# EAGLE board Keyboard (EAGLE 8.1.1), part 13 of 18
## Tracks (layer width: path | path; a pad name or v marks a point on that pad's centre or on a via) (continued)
S$13256 (continued)
  Bottom 0: 115.9,40.92 115.77,41.25
S$13257
  Bottom 0: 115.77,41.25 115.57,41.53
S$13258
  Bottom 0: 115.57,41.53 115.3,41.76
S$13259
  Bottom 0: 115.3,41.76 114.98,41.91
S$13260
  Bottom 0: 114.98,41.91 114.64,41.97
S$13261
  Bottom 0: 114.64,41.97 114.29,41.95
S$13262
  Bottom 0: 114.29,41.95 113.96,41.84
S$13263
  Bottom 0: 113.96,41.84 113.93,41.83
S$13264
  Bottom 0: 113.93,41.83 113.36,42.4
S$13265
  Bottom 0: 113.36,42.4 113.31,42.43
S$13266
  Bottom 0: 113.31,42.43 113.25,42.48
S$13267
  Bottom 0: 113.25,42.48 113.19,42.5
S$13268
  Bottom 0: 113.19,42.5 113.12,42.52
S$13269
  Bottom 0: 113.12,42.52 113.05,42.52
S$13270
  Bottom 0: 113.05,42.52 108.48,42.52
S$13271
  Bottom 0: 108.48,42.52 108.42,42.65
S$13272
  Bottom 0: 108.42,42.65 108.21,42.87
S$13273
  Bottom 0: 108.21,42.87 107.95,43.02
S$13274
  Bottom 0: 107.95,43.02 107.65,43.09
S$13275
  Bottom 0: 107.65,43.09 107.35,43.07
S$13276
  Bottom 0: 107.35,43.07 107.07,42.96
S$13277
  Bottom 0: 107.07,42.96 106.83,42.77
S$13278
  Bottom 0: 106.83,42.77 106.66,42.52
S$13279
  Bottom 0: 106.66,42.52 106.57,42.23
S$13280
  Bottom 0: 106.57,42.23 106.57,41.92
S$13281
  Bottom 0: 106.57,41.92 106.66,41.64
S$13282
  Bottom 0: 106.66,41.64 106.83,41.39
S$13283
  Bottom 0: 106.83,41.39 107.07,41.2
S$13284
  Bottom 0: 107.07,41.2 107.35,41.09
S$13285
  Bottom 0: 107.35,41.09 107.65,41.07
S$13286
  Bottom 0: 107.65,41.07 107.95,41.13
S$13287
  Bottom 0: 107.95,41.13 108.21,41.28
S$13288
  Bottom 0: 108.21,41.28 108.42,41.51
S$13289
  Bottom 0: 108.42,41.51 108.48,41.64
S$13290
  Bottom 0: 108.48,41.64 112.86,41.64
S$13291
  Bottom 0: 112.86,41.64 113.31,41.19
S$13292
  Bottom 0: 113.31,41.19 113.25,41.09
S$13293
  Bottom 0: 113.25,41.09 113.17,40.75
S$13294
  Bottom 0: 113.17,40.75 113.17,40.4
S$13295
  Bottom 0: 113.17,40.4 113.25,40.06
S$13296
  Bottom 0: 113.25,40.06 113.42,39.75
S$13297
  Bottom 0: 113.42,39.75 113.66,39.5
S$13298
  Bottom 0: 113.66,39.5 113.96,39.31
S$13299
  Bottom 0: 113.96,39.31 114.29,39.2
S$13300
  Bottom 0: 114.29,39.2 114.64,39.19
S$13301
  Bottom 0: 114.64,39.19 114.84,39.22
S$13302
  Bottom 0: 114.84,39.22 112.44,36.82
S$13303
  Bottom 0: 112.44,36.82 110.82,36.82
S$13304
  Bottom 0: 110.82,36.82 110.75,36.82
S$13305
  Bottom 0: 110.75,36.82 110.69,36.8
S$13306
  Bottom 0: 110.69,36.8 110.62,36.78
S$13307
  Bottom 0: 110.62,36.78 110.56,36.74
S$13308
  Bottom 0: 110.56,36.74 110.51,36.7
S$13309
  Bottom 0: 110.51,36.7 107.24,33.43
S$13310
  Bottom 0: 107.24,33.43 107.2,33.37
S$13311
  Bottom 0: 107.2,33.37 107.16,33.31
S$13312
  Bottom 0: 107.16,33.31 107.14,33.25
S$13313
  Bottom 0: 107.14,33.25 107.12,33.19
S$13314
  Bottom 0: 107.12,33.19 107.11,33.11
S$13315
  Bottom 0: 107.11,33.11 107.11,32.83
S$13316
  Bottom 0: 107.11,32.83 106.74,32.83
S$13317
  Bottom 0: 106.74,32.83 106.74,32.96
S$13318
  Bottom 0: 106.74,32.96 106.68,33.18
S$13319
  Bottom 0: 106.68,33.18 106.52,33.34
S$13320
  Bottom 0: 106.52,33.34 106.3,33.4
S$13321
  Bottom 0: 106.3,33.4 105.95,33.4
S$13322
  Bottom 0: 105.95,33.4 104.86,34.49
S$13323
  Bottom 0: 104.86,34.49 104.92,34.62
S$13324
  Bottom 0: 104.92,34.62 104.97,34.94
S$13325
  Bottom 0: 104.97,34.94 104.92,35.26
S$13326
  Bottom 0: 104.92,35.26 104.79,35.56
S$13327
  Bottom 0: 104.79,35.56 104.58,35.82
S$13328
  Bottom 0: 104.58,35.82 104.32,36.01
S$13329
  Bottom 0: 104.32,36.01 104.02,36.11
S$13330
  Bottom 0: 104.02,36.11 103.69,36.13
S$13331
  Bottom 0: 103.69,36.13 103.37,36.06
S$13332
  Bottom 0: 103.37,36.06 103.08,35.92
S$13333
  Bottom 0: 103.08,35.92 102.85,35.7
S$13334
  Bottom 0: 102.85,35.7 102.67,35.42
S$13335
  Bottom 0: 102.67,35.42 102.59,35.1
S$13336
  Bottom 0: 102.59,35.1 102.59,34.78
S$13337
  Bottom 0: 102.59,34.78 102.67,34.47
S$13338
  Bottom 0: 102.67,34.47 102.85,34.19
S$13339
  Bottom 0: 102.85,34.19 103.08,33.97
S$13340
  Bottom 0: 103.08,33.97 103.37,33.82
S$13341
  Bottom 0: 103.37,33.82 103.69,33.75
S$13342
  Bottom 0: 103.69,33.75 104.02,33.77
S$13343
  Bottom 0: 104.02,33.77 104.23,33.85
S$13344
  Bottom 0: 104.23,33.85 105.29,32.79
S$13345
  Bottom 0: 105.29,32.79 105.26,32.78
S$13346
  Bottom 0: 105.26,32.78 105.21,32.72
S$13347
  Bottom 0: 105.21,32.72 105.17,32.65
S$13348
  Bottom 0: 105.17,32.65 105.16,32.58
S$13349
  Bottom 0: 105.16,32.58 105.16,30.8
S$13350
  Bottom 0: 105.16,30.8 105.17,30.72
S$13351
  Bottom 0: 105.17,30.72 105.21,30.65
S$13352
  Bottom 0: 105.21,30.65 105.26,30.59
S$13353
  Bottom 0: 105.26,30.59 105.34,30.55
S$13354
  Bottom 0: 105.34,30.55 105.41,30.54
S$13355
  Bottom 0: 105.41,30.54 106.93,30.54
S$13356
  Bottom 0: 106.93,30.54 104.68,28.29
S$13357
  Bottom 0: 104.68,28.29 104.44,28.27
S$13358
  Bottom 0: 104.44,28.27 104.22,28.16
S$13359
  Bottom 0: 104.22,28.16 104.05,27.97
S$13360
  Bottom 0: 104.05,27.97 103.95,27.74
S$13361
  Bottom 0: 103.95,27.74 103.95,27.48
S$13362
  Bottom 0: 103.95,27.48 104.05,27.25
S$13363
  Bottom 0: 104.05,27.25 104.22,27.06
S$13364
  Bottom 0: 104.22,27.06 104.44,26.95
S$13365
  Bottom 0: 104.44,26.95 104.69,26.93
S$13366
  Bottom 0: 104.69,26.93 104.94,27
S$13367
  Bottom 0: 104.94,27 105.14,27.15
S$13368
  Bottom 0: 105.14,27.15 105.27,27.36
S$13369
  Bottom 0: 105.27,27.36 105.32,27.61
S$13370
  Bottom 0: 105.32,27.61 105.31,27.66
S$13371
  Bottom 0: 105.31,27.66 107.87,30.22
S$13372
  Bottom 0: 107.87,30.22 107.91,30.28
S$13373
  Bottom 0: 107.91,30.28 107.95,30.34
S$13374
  Bottom 0: 107.95,30.34 107.98,30.4
S$13375
  Bottom 0: 107.98,30.4 107.99,30.47
S$13376
  Bottom 0: 107.99,30.47 108,30.54
S$13377
  Bottom 0: 108,30.54 108,30.93
S$13378
  Bottom 0: 108,30.93 108.09,30.82
S$13379
  Bottom 0: 108.09,30.82 108.37,30.64
S$13380
  Bottom 0: 108.37,30.64 108.68,30.55
S$13381
  Bottom 0: 108.68,30.55 109,30.55
S$13382
  Bottom 0: 109,30.55 109.31,30.64
S$13383
  Bottom 0: 109.31,30.64 109.59,30.82
S$13384
  Bottom 0: 109.59,30.82 109.8,31.07
S$13385
  Bottom 0: 109.8,31.07 109.94,31.37
S$13386
  Bottom 0: 109.94,31.37 109.98,31.69
S$13387
  Bottom 0: 109.98,31.69 109.94,32.01
S$13388
  Bottom 0: 109.94,32.01 109.8,32.31
S$13389
  Bottom 0: 109.8,32.31 109.59,32.55
S$13390
  Bottom 0: 109.59,32.55 109.31,32.73
S$13391
  Bottom 0: 109.31,32.73 109,32.82
S$13392
  Bottom 0: 109,32.82 108.68,32.82
S$13393
  Bottom 0: 108.68,32.82 108.37,32.73
S$13394
  Bottom 0: 108.37,32.73 108.09,32.55
S$13395
  Bottom 0: 108.09,32.55 108,32.44
S$13396
  Bottom 0: 108,32.44 108,32.93
S$13397
  Bottom 0: 108,32.93 110.22,35.15
S$13398
  Bottom 0: 110.22,35.15 110.21,35.1
S$13399
  Bottom 0: 110.21,35.1 110.21,34.78
S$13400
  Bottom 0: 110.21,34.78 110.29,34.47
S$13401
  Bottom 0: 110.29,34.47 110.47,34.19
S$13402
  Bottom 0: 110.47,34.19 110.7,33.97
S$13403
  Bottom 0: 110.7,33.97 110.82,33.91
S$13404
  Bottom 0: 110.82,33.91 110.82,26.95
S$13405
  Bottom 0: 110.82,26.95 109.72,25.85
S$13406
  Bottom 0: 107.65,48.69 107.95,48.76
S$13407
  Bottom 0: 107.95,48.76 108.21,48.91
S$13408
  Bottom 0: 108.21,48.91 108.42,49.13
S$13409
  Bottom 0: 108.42,49.13 108.55,49.4
S$13410
  Bottom 0: 108.55,49.4 108.59,49.7
S$13411
  Bottom 0: 108.59,49.7 108.55,50
S$13412
  Bottom 0: 108.55,50 108.42,50.27
S$13413
  Bottom 0: 108.42,50.27 108.21,50.49
S$13414
  Bottom 0: 108.21,50.49 107.95,50.65
S$13415
  Bottom 0: 107.95,50.65 107.65,50.71
S$13416
  Bottom 0: 107.65,50.71 107.35,50.69
S$13417
  Bottom 0: 107.35,50.69 107.07,50.58
S$13418
  Bottom 0: 107.07,50.58 106.83,50.39
S$13419
  Bottom 0: 106.83,50.39 106.66,50.14
S$13420
  Bottom 0: 106.66,50.14 106.57,49.85
S$13421
  Bottom 0: 106.57,49.85 106.57,49.55
S$13422
  Bottom 0: 106.57,49.55 106.66,49.26
S$13423
  Bottom 0: 106.66,49.26 106.83,49.01
S$13424
  Bottom 0: 106.83,49.01 107.07,48.82
S$13425
  Bottom 0: 107.07,48.82 107.35,48.71
S$13426
  Bottom 0: 107.35,48.71 107.65,48.69
S$13427
  Bottom 0: 147.88,27.16 147.78,27.48
S$13428
  Bottom 0: 147.78,27.48 147.57,27.88
S$13429
  Bottom 0: 147.57,27.88 147.28,28.22
S$13430
  Bottom 0: 147.28,28.22 146.94,28.51
S$13431
  Bottom 0: 146.94,28.51 146.54,28.72
S$13432
  Bottom 0: 146.54,28.72 146.11,28.85
S$13433
  Bottom 0: 146.11,28.85 145.67,28.89
S$13434
  Bottom 0: 145.67,28.89 145.22,28.85
S$13435
  Bottom 0: 145.22,28.85 144.79,28.72
S$13436
  Bottom 0: 144.79,28.72 144.74,28.69
S$13437
  Bottom 0: 144.74,28.69 146.64,30.59
S$13438
  Bottom 0: 146.64,30.59 146.77,30.55
S$13439
  Bottom 0: 146.77,30.55 147.1,30.55
S$13440
  Bottom 0: 147.1,30.55 147.41,30.64
S$13441
  Bottom 0: 147.41,30.64 147.68,30.82
S$13442
  Bottom 0: 147.68,30.82 147.88,31.04
S$13443
  Bottom 0: 147.88,31.04 147.88,27.16
S$13444
  Bottom 0: 142.43,27.99 138.07,32.35
S$13445
  Bottom 0: 138.07,32.35 138.01,32.41
S$13446
  Bottom 0: 138.01,32.41 137.93,32.45
S$13447
  Bottom 0: 137.93,32.45 137.85,32.49
S$13448
  Bottom 0: 137.85,32.49 137.76,32.51
S$13449
  Bottom 0: 137.76,32.51 137.67,32.52
S$13450
  Bottom 0: 137.67,32.52 128.66,32.52
S$13451
  Bottom 0: 128.66,32.52 128.63,32.55
S$13452
  Bottom 0: 128.63,32.55 128.36,32.73
S$13453
  Bottom 0: 128.36,32.73 128.05,32.82
S$13454
  Bottom 0: 128.05,32.82 127.72,32.82
S$13455
  Bottom 0: 127.72,32.82 127.41,32.73
S$13456
  Bottom 0: 127.41,32.73 127.14,32.55
S$13457
  Bottom 0: 127.14,32.55 126.93,32.31
S$13458
  Bottom 0: 126.93,32.31 126.79,32.01
S$13459
  Bottom 0: 126.79,32.01 126.74,31.69
S$13460
  Bottom 0: 126.74,31.69 126.79,31.37
S$13461
  Bottom 0: 126.79,31.37 126.93,31.07
S$13462
  Bottom 0: 126.93,31.07 127.14,30.82
S$13463
  Bottom 0: 127.14,30.82 127.32,30.71
S$13464
  Bottom 0: 127.32,30.71 126.47,30.71
S$13465
  Bottom 0: 126.47,30.71 126.48,30.72
S$13466
  Bottom 0: 126.48,30.72 126.49,30.8
S$13467
  Bottom 0: 126.49,30.8 126.49,32.58
S$13468
  Bottom 0: 126.49,32.58 126.48,32.65
S$13469
  Bottom 0: 126.48,32.65 126.44,32.72
S$13470
  Bottom 0: 126.44,32.72 126.38,32.78
S$13471
  Bottom 0: 126.38,32.78 126.31,32.82
S$13472
  Bottom 0: 126.31,32.82 126.23,32.83
S$13473
  Bottom 0: 126.23,32.83 125.79,32.83
S$13474
  Bottom 0: 125.79,32.83 125.79,32.96
S$13475
  Bottom 0: 125.79,32.96 125.73,33.18
S$13476
  Bottom 0: 125.73,33.18 125.56,33.34
S$13477
  Bottom 0: 125.56,33.34 125.35,33.4
S$13478
  Bottom 0: 125.35,33.4 125,33.4
S$13479
  Bottom 0: 125,33.4 123.91,34.49
S$13480
  Bottom 0: 123.91,34.49 123.97,34.62
S$13481
  Bottom 0: 123.97,34.62 124.02,34.94
S$13482
  Bottom 0: 124.02,34.94 123.97,35.26
S$13483
  Bottom 0: 123.97,35.26 123.84,35.56
S$13484
  Bottom 0: 123.84,35.56 123.64,35.82
S$13485
  Bottom 0: 123.64,35.82 123.37,36.01
S$13486
  Bottom 0: 123.37,36.01 123.07,36.11
S$13487
  Bottom 0: 123.07,36.11 122.74,36.13
S$13488
  Bottom 0: 122.74,36.13 122.42,36.06
S$13489
  Bottom 0: 122.42,36.06 122.13,35.92
S$13490
  Bottom 0: 122.13,35.92 121.9,35.7
S$13491
  Bottom 0: 121.9,35.7 121.72,35.42
S$13492
  Bottom 0: 121.72,35.42 121.64,35.1
S$13493
  Bottom 0: 121.64,35.1 121.64,34.78
S$13494
  Bottom 0: 121.64,34.78 121.72,34.47
S$13495
  Bottom 0: 121.72,34.47 121.9,34.19
S$13496
  Bottom 0: 121.9,34.19 122.13,33.97
S$13497
  Bottom 0: 122.13,33.97 122.42,33.82
S$13498
  Bottom 0: 122.42,33.82 122.74,33.75
S$13499
  Bottom 0: 122.74,33.75 123.07,33.77
S$13500
  Bottom 0: 123.07,33.77 123.28,33.85
S$13501
  Bottom 0: 123.28,33.85 124.34,32.79
S$13502
  Bottom 0: 124.34,32.79 124.31,32.78
S$13503
  Bottom 0: 124.31,32.78 124.25,32.72
S$13504
  Bottom 0: 124.25,32.72 124.21,32.65
S$13505
  Bottom 0: 124.21,32.65 124.2,32.58
S$13506
  Bottom 0: 124.2,32.58 124.2,30.8
S$13507
  Bottom 0: 124.2,30.8 124.21,30.72
S$13508
  Bottom 0: 124.21,30.72 124.22,30.71
S$13509
  Bottom 0: 124.22,30.71 118.11,30.71
S$13510
  Bottom 0: 118.11,30.71 118.07,30.95
S$13511
  Bottom 0: 118.07,30.95 117.94,31.22
S$13512
  Bottom 0: 117.94,31.22 117.74,31.44
S$13513
  Bottom 0: 117.74,31.44 117.47,31.59
S$13514
  Bottom 0: 117.47,31.59 117.18,31.66
S$13515
  Bottom 0: 117.18,31.66 117.13,31.66
S$13516
  Bottom 0: 117.13,31.66 123.99,38.52
S$13517
  Bottom 0: 123.99,38.52 138,38.52
S$13518
  Bottom 0: 138,38.52 138.07,38.52
S$13519
  Bottom 0: 138.07,38.52 138.13,38.54
S$13520
  Bottom 0: 138.13,38.54 138.19,38.56
S$13521
  Bottom 0: 138.19,38.56 138.25,38.6
S$13522
  Bottom 0: 138.25,38.6 138.31,38.65
S$13523
  Bottom 0: 138.31,38.65 149.63,49.96
S$13524
  Bottom 0: 149.63,49.96 149.65,49.99
S$13525
  Bottom 0: 149.65,49.99 149.65,48.39
S$13526
  Bottom 0: 149.65,48.39 144.18,42.92
S$13527
  Bottom 0: 144.18,42.92 144.14,42.87
S$13528
  Bottom 0: 144.14,42.87 144.1,42.81
S$13529
  Bottom 0: 144.1,42.81 144.08,42.75
S$13530
  Bottom 0: 144.08,42.75 144.06,42.68
S$13531
  Bottom 0: 144.06,42.68 144.06,42.61
S$13532
  Bottom 0: 144.06,42.61 144.06,38.52
S$13533
  Bottom 0: 144.06,38.52 144.06,38.45
S$13534
  Bottom 0: 144.06,38.45 144.08,38.38
S$13535
  Bottom 0: 144.08,38.38 144.1,38.32
S$13536
  Bottom 0: 144.1,38.32 144.14,38.26
S$13537
  Bottom 0: 144.14,38.26 144.18,38.2
S$13538
  Bottom 0: 144.18,38.2 145.28,37.11
S$13539
  Bottom 0: 145.28,37.11 145.28,36.93
S$13540
  Bottom 0: 145.28,36.93 145.36,36.7
S$13541
  Bottom 0: 145.36,36.7 145.54,36.51
S$13542
  Bottom 0: 145.54,36.51 145.76,36.4
S$13543
  Bottom 0: 145.76,36.4 146.01,36.38
S$13544
  Bottom 0: 146.01,36.38 146.25,36.45
S$13545
  Bottom 0: 146.25,36.45 146.37,36.53
S$13546
  Bottom 0: 146.37,36.53 146.37,32.67
S$13547
  Bottom 0: 146.37,32.67 146.19,32.55
S$13548
  Bottom 0: 146.19,32.55 145.98,32.31
S$13549
  Bottom 0: 145.98,32.31 145.84,32.01
S$13550
  Bottom 0: 145.84,32.01 145.79,31.69
S$13551
  Bottom 0: 145.79,31.69 145.83,31.39
S$13552
  Bottom 0: 145.83,31.39 145.54,31.09
S$13553
  Bottom 0: 145.54,31.09 145.54,32.58
S$13554
  Bottom 0: 145.54,32.58 145.53,32.65
S$13555
  Bottom 0: 145.53,32.65 145.49,32.72
S$13556
  Bottom 0: 145.49,32.72 145.43,32.78
S$13557
  Bottom 0: 145.43,32.78 145.36,32.82
S$13558
  Bottom 0: 145.36,32.82 145.28,32.83
S$13559
  Bottom 0: 145.28,32.83 144.84,32.83
S$13560
  Bottom 0: 144.84,32.83 144.84,32.96
S$13561
  Bottom 0: 144.84,32.96 144.78,33.18
S$13562
  Bottom 0: 144.78,33.18 144.62,33.34
S$13563
  Bottom 0: 144.62,33.34 144.4,33.4
S$13564
  Bottom 0: 144.4,33.4 144.04,33.4
S$13565
  Bottom 0: 144.04,33.4 142.96,34.48
S$13566
  Bottom 0: 142.96,34.48 143.02,34.62
S$13567
  Bottom 0: 143.02,34.62 143.06,34.94
S$13568
  Bottom 0: 143.06,34.94 143.02,35.26
S$13569
  Bottom 0: 143.02,35.26 142.89,35.56
S$13570
  Bottom 0: 142.89,35.56 142.69,35.81
S$13571
  Bottom 0: 142.69,35.81 142.42,36
S$13572
  Bottom 0: 142.42,36 142.12,36.11
S$13573
  Bottom 0: 142.12,36.11 141.79,36.13
S$13574
  Bottom 0: 141.79,36.13 141.47,36.06
S$13575
  Bottom 0: 141.47,36.06 141.18,35.91
S$13576
  Bottom 0: 141.18,35.91 140.95,35.69
S$13577
  Bottom 0: 140.95,35.69 140.77,35.41
S$13578
  Bottom 0: 140.77,35.41 140.69,35.1
S$13579
  Bottom 0: 140.69,35.1 140.69,34.77
S$13580
  Bottom 0: 140.69,34.77 140.77,34.46
S$13581
  Bottom 0: 140.77,34.46 140.95,34.19
S$13582
  Bottom 0: 140.95,34.19 141.18,33.96
S$13583
  Bottom 0: 141.18,33.96 141.47,33.81
S$13584
  Bottom 0: 141.47,33.81 141.79,33.75
S$13585
  Bottom 0: 141.79,33.75 142.12,33.77
S$13586
  Bottom 0: 142.12,33.77 142.33,33.85
S$13587
  Bottom 0: 142.33,33.85 143.39,32.79
S$13588
  Bottom 0: 143.39,32.79 143.36,32.78
S$13589
  Bottom 0: 143.36,32.78 143.3,32.72
S$13590
  Bottom 0: 143.3,32.72 143.26,32.65
S$13591
  Bottom 0: 143.26,32.65 143.25,32.58
S$13592
  Bottom 0: 143.25,32.58 143.25,30.8
S$13593
  Bottom 0: 143.25,30.8 143.26,30.72
S$13594
  Bottom 0: 143.26,30.72 143.3,30.65
S$13595
  Bottom 0: 143.3,30.65 143.36,30.59
S$13596
  Bottom 0: 143.36,30.59 143.43,30.55
S$13597
  Bottom 0: 143.43,30.55 143.51,30.54
S$13598
  Bottom 0: 143.51,30.54 144.99,30.54
S$13599
  Bottom 0: 144.99,30.54 142.43,27.99
S$13600
  Bottom 0: 130.36,33.75 130.69,33.77
S$13601
  Bottom 0: 130.69,33.77 130.99,33.88
S$13602
  Bottom 0: 130.99,33.88 131.25,34.07
S$13603
  Bottom 0: 131.25,34.07 131.46,34.32
S$13604
  Bottom 0: 131.46,34.32 131.59,34.62
S$13605
  Bottom 0: 131.59,34.62 131.64,34.94
S$13606
  Bottom 0: 131.64,34.94 131.59,35.26
S$13607
  Bottom 0: 131.59,35.26 131.46,35.56
S$13608
  Bottom 0: 131.46,35.56 131.25,35.82
S$13609
  Bottom 0: 131.25,35.82 130.99,36.01
S$13610
  Bottom 0: 130.99,36.01 130.69,36.11
S$13611
  Bottom 0: 130.69,36.11 130.36,36.13
S$13612
  Bottom 0: 130.36,36.13 130.04,36.06
S$13613
  Bottom 0: 130.04,36.06 129.75,35.92
S$13614
  Bottom 0: 129.75,35.92 129.52,35.7
S$13615
  Bottom 0: 129.52,35.7 129.34,35.42
S$13616
  Bottom 0: 129.34,35.42 129.26,35.1
S$13617
  Bottom 0: 129.26,35.1 129.26,34.78
S$13618
  Bottom 0: 129.26,34.78 129.34,34.47
S$13619
  Bottom 0: 129.34,34.47 129.52,34.19
S$13620
  Bottom 0: 129.52,34.19 129.75,33.97
S$13621
  Bottom 0: 129.75,33.97 130.04,33.82
S$13622
  Bottom 0: 130.04,33.82 130.36,33.75
S$13623
  Bottom 0: 90.4,30.74 90.53,30.82
S$13624
  Bottom 0: 90.53,30.82 90.75,31.07
S$13625
  Bottom 0: 90.75,31.07 90.88,31.37
S$13626
  Bottom 0: 90.88,31.37 90.93,31.69
S$13627
  Bottom 0: 90.93,31.69 90.88,32.01
S$13628
  Bottom 0: 90.88,32.01 90.75,32.31
S$13629
  Bottom 0: 90.75,32.31 90.53,32.55
S$13630
  Bottom 0: 90.53,32.55 90.36,32.67
S$13631
  Bottom 0: 90.36,32.67 90.36,41.16
S$13632
  Bottom 0: 90.36,41.16 91.55,42.34
S$13633
  Bottom 0: 91.55,42.34 91.58,42.34
S$13634
  Bottom 0: 91.58,42.34 91.66,42.37
S$13635
  Bottom 0: 91.66,42.37 91.74,42.4
S$13636
  Bottom 0: 91.74,42.4 91.82,42.45
S$13637
  Bottom 0: 91.82,42.45 91.89,42.51
S$13638
  Bottom 0: 91.89,42.51 95.95,46.58
S$13639
  Bottom 0: 95.95,46.58 95.93,46.53
S$13640
  Bottom 0: 95.93,46.53 95.8,46.1
S$13641
  Bottom 0: 95.8,46.1 95.75,45.66
S$13642
  Bottom 0: 95.75,45.66 95.8,45.21
S$13643
  Bottom 0: 95.8,45.21 95.93,44.78
S$13644
  Bottom 0: 95.93,44.78 96.14,44.39
S$13645
  Bottom 0: 96.14,44.39 96.43,44.04
S$13646
  Bottom 0: 96.43,44.04 96.77,43.76
S$13647
  Bottom 0: 96.77,43.76 97.17,43.54
S$13648
  Bottom 0: 97.17,43.54 97.59,43.42
S$13649
  Bottom 0: 97.59,43.42 98.04,43.37
S$13650
  Bottom 0: 98.04,43.37 98.49,43.42
S$13651
  Bottom 0: 98.49,43.42 98.91,43.54
S$13652
  Bottom 0: 98.91,43.54 99.31,43.76
S$13653
  Bottom 0: 99.31,43.76 99.66,44.04
S$13654
  Bottom 0: 99.66,44.04 99.94,44.39
S$13655
  Bottom 0: 99.94,44.39 100.15,44.78
S$13656
  Bottom 0: 100.15,44.78 100.28,45.21
S$13657
  Bottom 0: 100.28,45.21 100.33,45.66
S$13658
  Bottom 0: 100.33,45.66 100.28,46.1
S$13659
  Bottom 0: 100.28,46.1 100.15,46.53
S$13660
  Bottom 0: 100.15,46.53 99.94,46.93
S$13661
  Bottom 0: 99.94,46.93 99.66,47.27
S$13662
  Bottom 0: 99.66,47.27 99.31,47.56
S$13663
  Bottom 0: 99.31,47.56 98.91,47.77
S$13664
  Bottom 0: 98.91,47.77 98.49,47.89
S$13665
  Bottom 0: 98.49,47.89 98.04,47.94
S$13666
  Bottom 0: 98.04,47.94 97.59,47.89
S$13667
  Bottom 0: 97.59,47.89 97.17,47.77
S$13668
  Bottom 0: 97.17,47.77 97.12,47.74
S$13669
  Bottom 0: 97.12,47.74 99.02,49.64
S$13670
  Bottom 0: 99.02,49.64 99.15,49.6
S$13671
  Bottom 0: 99.15,49.6 99.47,49.6
S$13672
  Bottom 0: 99.47,49.6 99.78,49.7
S$13673
  Bottom 0: 99.78,49.7 100.06,49.87
S$13674
  Bottom 0: 100.06,49.87 100.27,50.11
S$13675
  Bottom 0: 100.27,50.11 100.41,50.42
S$13676
  Bottom 0: 100.41,50.42 100.45,50.74
S$13677
  Bottom 0: 100.45,50.74 100.45,50.75
S$13678
  Bottom 0: 100.45,50.75 101.41,49.79
S$13679
  Bottom 0: 101.41,49.79 101.41,44.43
S$13680
  Bottom 0: 101.41,44.43 101.26,44.38
S$13681
  Bottom 0: 101.26,44.38 100.96,44.19
S$13682
  Bottom 0: 100.96,44.19 100.72,43.94
S$13683
  Bottom 0: 100.72,43.94 100.55,43.63
S$13684
  Bottom 0: 100.55,43.63 100.47,43.29
S$13685
  Bottom 0: 100.47,43.29 100.47,42.94
S$13686
  Bottom 0: 100.47,42.94 100.55,42.6
S$13687
  Bottom 0: 100.55,42.6 100.72,42.29
S$13688
  Bottom 0: 100.72,42.29 100.96,42.04
S$13689
  Bottom 0: 100.96,42.04 101.26,41.85
S$13690
  Bottom 0: 101.26,41.85 101.59,41.74
S$13691
  Bottom 0: 101.59,41.74 101.94,41.73
S$13692
  Bottom 0: 101.94,41.73 102.13,41.76
S$13693
  Bottom 0: 102.13,41.76 95.81,35.44
S$13694
  Bottom 0: 95.81,35.44 95.8,35.45
S$13695
  Bottom 0: 95.8,35.45 95.72,35.48
S$13696
  Bottom 0: 95.72,35.48 95.63,35.5
S$13697
  Bottom 0: 95.63,35.5 95.54,35.51
S$13698
  Bottom 0: 95.54,35.51 93.38,35.51
S$13699
  Bottom 0: 93.38,35.51 93.36,35.56
S$13700
  Bottom 0: 93.36,35.56 93.15,35.81
S$13701
  Bottom 0: 93.15,35.81 92.89,36
S$13702
  Bottom 0: 92.89,36 92.58,36.11
S$13703
  Bottom 0: 92.58,36.11 92.25,36.13
S$13704
  Bottom 0: 92.25,36.13 91.94,36.06
S$13705
  Bottom 0: 91.94,36.06 91.64,35.91
S$13706
  Bottom 0: 91.64,35.91 91.41,35.69
S$13707
  Bottom 0: 91.41,35.69 91.24,35.41
S$13708
  Bottom 0: 91.24,35.41 91.15,35.1
S$13709
  Bottom 0: 91.15,35.1 91.15,34.77
S$13710
  Bottom 0: 91.15,34.77 91.24,34.46
S$13711
  Bottom 0: 91.24,34.46 91.41,34.19
S$13712
  Bottom 0: 91.41,34.19 91.64,33.96
S$13713
  Bottom 0: 91.64,33.96 91.94,33.81
S$13714
  Bottom 0: 91.94,33.81 92.25,33.75
S$13715
  Bottom 0: 92.25,33.75 92.58,33.77
S$13716
  Bottom 0: 92.58,33.77 92.89,33.88
S$13717
  Bottom 0: 92.89,33.88 93.15,34.06
S$13718
  Bottom 0: 93.15,34.06 93.36,34.32
S$13719
  Bottom 0: 93.36,34.32 93.38,34.37
S$13720
  Bottom 0: 93.38,34.37 95.3,34.37
S$13721
  Bottom 0: 95.3,34.37 95.42,34.25
S$13722
  Bottom 0: 95.42,34.25 98.02,31.66
S$13723
  Bottom 0: 98.02,31.66 97.82,31.64
S$13724
  Bottom 0: 97.82,31.64 97.54,31.53
S$13725
  Bottom 0: 97.54,31.53 97.31,31.34
S$13726
  Bottom 0: 97.31,31.34 97.14,31.09
S$13727
  Bottom 0: 97.14,31.09 97.05,30.8
S$13728
  Bottom 0: 97.05,30.8 97.05,30.74
S$13729
  Bottom 0: 97.05,30.74 90.4,30.74
S$13730
  Bottom 0: 95.59,39.19 95.93,39.25
S$13731
  Bottom 0: 95.93,39.25 96.25,39.4
S$13732
  Bottom 0: 96.25,39.4 96.52,39.62
S$13733
  Bottom 0: 96.52,39.62 96.72,39.91
S$13734
  Bottom 0: 96.72,39.91 96.85,40.23
S$13735
  Bottom 0: 96.85,40.23 96.9,40.58
S$13736
  Bottom 0: 96.9,40.58 96.85,40.92
S$13737
  Bottom 0: 96.85,40.92 96.72,41.25
S$13738
  Bottom 0: 96.72,41.25 96.52,41.53
S$13739
  Bottom 0: 96.52,41.53 96.25,41.76
S$13740
  Bottom 0: 96.25,41.76 95.93,41.91
S$13741
  Bottom 0: 95.93,41.91 95.59,41.97
S$13742
  Bottom 0: 95.59,41.97 95.24,41.95
S$13743
  Bottom 0: 95.24,41.95 94.91,41.84
S$13744
  Bottom 0: 94.91,41.84 94.61,41.65
S$13745
  Bottom 0: 94.61,41.65 94.37,41.4
S$13746
  Bottom 0: 94.37,41.4 94.2,41.09
S$13747
  Bottom 0: 94.2,41.09 94.11,40.75
S$13748
  Bottom 0: 94.11,40.75 94.11,40.4
S$13749
  Bottom 0: 94.11,40.4 94.2,40.06
S$13750
  Bottom 0: 94.2,40.06 94.37,39.75
S$13751
  Bottom 0: 94.37,39.75 94.61,39.5
S$13752
  Bottom 0: 94.61,39.5 94.91,39.31
S$13753
  Bottom 0: 94.91,39.31 95.24,39.2
S$13754
  Bottom 0: 95.24,39.2 95.59,39.19
S$13755
  Bottom 0: 186.02,32.26 186,32.31
S$13756
  Bottom 0: 186,32.31 185.78,32.55
S$13757
  Bottom 0: 185.78,32.55 185.51,32.73
S$13758
  Bottom 0: 185.51,32.73 185.47,32.74
S$13759
  Bottom 0: 185.47,32.74 185.95,32.74
S$13760
  Bottom 0: 185.95,32.74 186.04,32.74
S$13761
  Bottom 0: 186.04,32.74 186.13,32.76
S$13762
  Bottom 0: 186.13,32.76 186.22,32.8
S$13763
  Bottom 0: 186.22,32.8 186.29,32.84
S$13764
  Bottom 0: 186.29,32.84 186.36,32.91
S$13765
  Bottom 0: 186.36,32.91 187.26,33.8
S$13766
  Bottom 0: 187.26,33.8 187.52,33.75
S$13767
  Bottom 0: 187.52,33.75 187.84,33.77
S$13768
  Bottom 0: 187.84,33.77 188.15,33.88
S$13769
  Bottom 0: 188.15,33.88 188.41,34.07
S$13770
  Bottom 0: 188.41,34.07 188.62,34.32
S$13771
  Bottom 0: 188.62,34.32 188.74,34.62
S$13772
  Bottom 0: 188.74,34.62 188.79,34.94
S$13773
  Bottom 0: 188.79,34.94 188.74,35.26
S$13774
  Bottom 0: 188.74,35.26 188.62,35.56
S$13775
  Bottom 0: 188.62,35.56 188.41,35.82
S$13776
  Bottom 0: 188.41,35.82 188.15,36.01
S$13777
  Bottom 0: 188.15,36.01 187.84,36.11
S$13778
  Bottom 0: 187.84,36.11 187.52,36.13
S$13779
  Bottom 0: 187.52,36.13 187.19,36.06
S$13780
  Bottom 0: 187.19,36.06 186.9,35.92
S$13781
  Bottom 0: 186.9,35.92 186.67,35.7
S$13782
  Bottom 0: 186.67,35.7 186.5,35.42
S$13783
  Bottom 0: 186.5,35.42 186.41,35.1
S$13784
  Bottom 0: 186.41,35.1 186.41,34.78
S$13785
  Bottom 0: 186.41,34.78 186.46,34.61
S$13786
  Bottom 0: 186.46,34.61 185.72,33.88
S$13787
  Bottom 0: 185.72,33.88 180.51,33.88
S$13788
  Bottom 0: 180.51,33.88 180.53,33.88
S$13789
  Bottom 0: 180.53,33.88 180.79,34.07
S$13790
  Bottom 0: 180.79,34.07 181,34.32
S$13791
  Bottom 0: 181,34.32 181.12,34.62
S$13792
  Bottom 0: 181.12,34.62 181.17,34.94
S$13793
  Bottom 0: 181.17,34.94 181.12,35.26
S$13794
  Bottom 0: 181.12,35.26 181,35.56
S$13795
  Bottom 0: 181,35.56 180.79,35.82
S$13796
  Bottom 0: 180.79,35.82 180.53,36.01
S$13797
  Bottom 0: 180.53,36.01 180.22,36.11
S$13798
  Bottom 0: 180.22,36.11 179.9,36.13
S$13799
  Bottom 0: 179.9,36.13 179.57,36.06
S$13800
  Bottom 0: 179.57,36.06 179.28,35.92
S$13801
  Bottom 0: 179.28,35.92 179.05,35.7
S$13802
  Bottom 0: 179.05,35.7 178.98,35.57
S$13803
  Bottom 0: 178.98,35.57 178.98,36.37
S$13804
  Bottom 0: 178.98,36.37 180.11,37.5
S$13805
  Bottom 0: 180.11,37.5 180.17,37.56
S$13806
  Bottom 0: 180.17,37.56 180.22,37.64
S$13807
  Bottom 0: 180.22,37.64 180.25,37.72
S$13808
  Bottom 0: 180.25,37.72 180.27,37.81
S$13809
  Bottom 0: 180.27,37.81 180.28,37.9
S$13810
  Bottom 0: 180.28,37.9 180.28,51.79
S$13811
  Bottom 0: 180.28,51.79 188.57,51.79
S$13812
  Bottom 0: 188.57,51.79 188.52,51.73
S$13813
  Bottom 0: 188.52,51.73 188.43,51.49
S$13814
  Bottom 0: 188.43,51.49 188.43,51.24
S$13815
  Bottom 0: 188.43,51.24 188.52,51
S$13816
  Bottom 0: 188.52,51 188.69,50.81
S$13817
  Bottom 0: 188.69,50.81 188.9,50.71
S$13818
  Bottom 0: 188.9,50.71 191.12,48.5
S$13819
  Bottom 0: 191.12,48.5 191.17,48.46
S$13820
  Bottom 0: 191.17,48.46 191.23,48.42
S$13821
  Bottom 0: 191.23,48.42 191.29,48.4
S$13822
  Bottom 0: 191.29,48.4 191.35,48.38
S$13823
  Bottom 0: 191.35,48.38 191.43,48.37
S$13824
  Bottom 0: 191.43,48.37 193.34,48.37
S$13825
  Bottom 0: 193.34,48.37 193.85,47.86
S$13826
  Bottom 0: 193.85,47.86 193.74,47.89
S$13827
  Bottom 0: 193.74,47.89 193.29,47.94
S$13828
  Bottom 0: 193.29,47.94 192.84,47.89
S$13829
  Bottom 0: 192.84,47.89 192.42,47.77
S$13830
  Bottom 0: 192.42,47.77 192.02,47.56
S$13831
  Bottom 0: 192.02,47.56 191.68,47.27
S$13832
  Bottom 0: 191.68,47.27 191.39,46.93
S$13833
  Bottom 0: 191.39,46.93 191.18,46.53
S$13834
  Bottom 0: 191.18,46.53 191.05,46.1
S$13835
  Bottom 0: 191.05,46.1 191,45.66
S$13836
  Bottom 0: 191,45.66 191.05,45.21
S$13837
  Bottom 0: 191.05,45.21 191.18,44.78
S$13838
  Bottom 0: 191.18,44.78 191.39,44.39
S$13839
  Bottom 0: 191.39,44.39 191.68,44.04
S$13840
  Bottom 0: 191.68,44.04 192.02,43.76
S$13841
  Bottom 0: 192.02,43.76 192.42,43.54
S$13842
  Bottom 0: 192.42,43.54 192.84,43.42
S$13843
  Bottom 0: 192.84,43.42 193.29,43.37
S$13844
  Bottom 0: 193.29,43.37 193.74,43.42
S$13845
  Bottom 0: 193.74,43.42 194.16,43.54
S$13846
  Bottom 0: 194.16,43.54 194.56,43.76
S$13847
  Bottom 0: 194.56,43.76 194.9,44.04
S$13848
  Bottom 0: 194.9,44.04 195.19,44.39
S$13849
  Bottom 0: 195.19,44.39 195.41,44.78
S$13850
  Bottom 0: 195.41,44.78 195.53,45.21
S$13851
  Bottom 0: 195.53,45.21 195.58,45.66
S$13852
  Bottom 0: 195.58,45.66 195.53,46.1
S$13853
  Bottom 0: 195.53,46.1 195.5,46.22
S$13854
  Bottom 0: 195.5,46.22 196.66,45.06
S$13855
  Bottom 0: 196.66,45.06 196.66,44.43
S$13856
  Bottom 0: 196.66,44.43 196.51,44.38
S$13857
  Bottom 0: 196.51,44.38 196.21,44.19
S$13858
  Bottom 0: 196.21,44.19 195.97,43.94
S$13859
  Bottom 0: 195.97,43.94 195.8,43.63
S$13860
  Bottom 0: 195.8,43.63 195.72,43.29
S$13861
  Bottom 0: 195.72,43.29 195.72,42.94
S$13862
  Bottom 0: 195.72,42.94 195.8,42.6
S$13863
  Bottom 0: 195.8,42.6 195.97,42.29
S$13864
  Bottom 0: 195.97,42.29 196.21,42.04
S$13865
  Bottom 0: 196.21,42.04 196.51,41.85
S$13866
  Bottom 0: 196.51,41.85 196.84,41.74
S$13867
  Bottom 0: 196.84,41.74 197.19,41.73
S$13868
  Bottom 0: 197.19,41.73 197.53,41.79
S$13869
  Bottom 0: 197.53,41.79 197.85,41.94
S$13870
  Bottom 0: 197.85,41.94 198.12,42.16
S$13871
  Bottom 0: 198.12,42.16 198.33,42.45
S$13872
  Bottom 0: 198.33,42.45 198.38,42.58
S$13873
  Bottom 0: 198.38,42.58 198.38,36.95
S$13874
  Bottom 0: 198.38,36.95 197.14,36.95
S$13875
  Bottom 0: 197.14,36.95 197.05,36.95
S$13876
  Bottom 0: 197.05,36.95 196.96,36.93
S$13877
  Bottom 0: 196.96,36.93 196.88,36.89
S$13878
  Bottom 0: 196.88,36.89 196.8,36.85
S$13879
  Bottom 0: 196.8,36.85 196.74,36.79
S$13880
  Bottom 0: 196.74,36.79 192.21,32.26
S$13881
  Bottom 0: 192.21,32.26 186.02,32.26
S$13882
  Bottom 0: 190.84,39.19 191.18,39.25
S$13883
  Bottom 0: 191.18,39.25 191.5,39.4
S$13884
  Bottom 0: 191.5,39.4 191.77,39.62
S$13885
  Bottom 0: 191.77,39.62 191.98,39.91
S$13886
  Bottom 0: 191.98,39.91 192.1,40.23
S$13887
  Bottom 0: 192.1,40.23 192.15,40.58
S$13888
  Bottom 0: 192.15,40.58 192.1,40.92
S$13889
  Bottom 0: 192.1,40.92 191.98,41.25
S$13890
  Bottom 0: 191.98,41.25 191.77,41.53
S$13891
  Bottom 0: 191.77,41.53 191.5,41.76
S$13892
  Bottom 0: 191.5,41.76 191.18,41.91
S$13893
  Bottom 0: 191.18,41.91 190.84,41.97
S$13894
  Bottom 0: 190.84,41.97 190.49,41.95
S$13895
  Bottom 0: 190.49,41.95 190.16,41.84
S$13896
  Bottom 0: 190.16,41.84 190.13,41.83
S$13897
  Bottom 0: 190.13,41.83 189.56,42.4
S$13898
  Bottom 0: 189.56,42.4 189.5,42.43
S$13899
  Bottom 0: 189.5,42.43 189.44,42.48
S$13900
  Bottom 0: 189.44,42.48 189.38,42.5
S$13901
  Bottom 0: 189.38,42.5 189.32,42.52
S$13902
  Bottom 0: 189.32,42.52 189.25,42.52
S$13903
  Bottom 0: 189.25,42.52 184.69,42.52
S$13904
  Bottom 0: 184.69,42.52 184.62,42.65
S$13905
  Bottom 0: 184.62,42.65 184.42,42.87
S$13906
  Bottom 0: 184.42,42.87 184.16,43.02
S$13907
  Bottom 0: 184.16,43.02 183.86,43.09
S$13908
  Bottom 0: 183.86,43.09 183.56,43.07
S$13909
  Bottom 0: 183.56,43.07 183.28,42.96
S$13910
  Bottom 0: 183.28,42.96 183.04,42.77
S$13911
  Bottom 0: 183.04,42.77 182.87,42.52
S$13912
  Bottom 0: 182.87,42.52 182.78,42.23
S$13913
  Bottom 0: 182.78,42.23 182.78,41.92
S$13914
  Bottom 0: 182.78,41.92 182.87,41.64
S$13915
  Bottom 0: 182.87,41.64 183.04,41.39
S$13916
  Bottom 0: 183.04,41.39 183.28,41.2
S$13917
  Bottom 0: 183.28,41.2 183.56,41.09
S$13918
  Bottom 0: 183.56,41.09 183.86,41.07
S$13919
  Bottom 0: 183.86,41.07 184.16,41.13
S$13920
  Bottom 0: 184.16,41.13 184.42,41.28
S$13921
  Bottom 0: 184.42,41.28 184.62,41.51
S$13922
  Bottom 0: 184.62,41.51 184.69,41.64
S$13923
  Bottom 0: 184.69,41.64 189.06,41.64
S$13924
  Bottom 0: 189.06,41.64 189.5,41.19
S$13925
  Bottom 0: 189.5,41.19 189.45,41.09
S$13926
  Bottom 0: 189.45,41.09 189.37,40.75
S$13927
  Bottom 0: 189.37,40.75 189.37,40.4
S$13928
  Bottom 0: 189.37,40.4 189.45,40.06
S$13929
  Bottom 0: 189.45,40.06 189.62,39.75
S$13930
  Bottom 0: 189.62,39.75 189.86,39.5
S$13931
  Bottom 0: 189.86,39.5 190.16,39.31
S$13932
  Bottom 0: 190.16,39.31 190.49,39.2
S$13933
  Bottom 0: 190.49,39.2 190.84,39.19
S$13934
  Bottom 0: 183.86,48.69 184.16,48.76
S$13935
  Bottom 0: 184.16,48.76 184.42,48.91
S$13936
  Bottom 0: 184.42,48.91 184.62,49.13
S$13937
  Bottom 0: 184.62,49.13 184.76,49.4
S$13938
  Bottom 0: 184.76,49.4 184.8,49.7
S$13939
  Bottom 0: 184.8,49.7 184.76,50
S$13940
  Bottom 0: 184.76,50 184.62,50.27
S$13941
  Bottom 0: 184.62,50.27 184.42,50.49
S$13942
  Bottom 0: 184.42,50.49 184.16,50.65
S$13943
  Bottom 0: 184.16,50.65 183.86,50.71
S$13944
  Bottom 0: 183.86,50.71 183.56,50.69
S$13945
  Bottom 0: 183.56,50.69 183.28,50.58
S$13946
  Bottom 0: 183.28,50.58 183.04,50.39
S$13947
  Bottom 0: 183.04,50.39 182.87,50.14
S$13948
  Bottom 0: 182.87,50.14 182.78,49.85
S$13949
  Bottom 0: 182.78,49.85 182.78,49.55
S$13950
  Bottom 0: 182.78,49.55 182.87,49.26
S$13951
  Bottom 0: 182.87,49.26 183.04,49.01
S$13952
  Bottom 0: 183.04,49.01 183.28,48.82
S$13953
  Bottom 0: 183.28,48.82 183.56,48.71
S$13954
  Bottom 0: 183.56,48.71 183.86,48.69
S$13955
  Bottom 0: 150.53,35.51 150.51,35.56
S$13956
  Bottom 0: 150.51,35.56 150.3,35.81
S$13957
  Bottom 0: 150.3,35.81 150.04,36
S$13958
  Bottom 0: 150.04,36 149.74,36.11
S$13959
  Bottom 0: 149.74,36.11 149.45,36.13
S$13960
  Bottom 0: 149.45,36.13 150.97,37.65
S$13961
  Bottom 0: 150.97,37.65 152.31,37.65
S$13962
  Bottom 0: 152.31,37.65 152.38,37.66
S$13963
  Bottom 0: 152.38,37.66 152.45,37.67
S$13964
  Bottom 0: 152.45,37.67 152.51,37.7
S$13965
  Bottom 0: 152.51,37.7 152.57,37.74
S$13966
  Bottom 0: 152.57,37.74 152.63,37.78
S$13967
  Bottom 0: 152.63,37.78 157.65,42.8
S$13968
  Bottom 0: 157.65,42.8 157.7,42.6
S$13969
  Bottom 0: 157.7,42.6 157.87,42.29
S$13970
  Bottom 0: 157.87,42.29 158.11,42.04
S$13971
  Bottom 0: 158.11,42.04 158.41,41.85
S$13972
  Bottom 0: 158.41,41.85 158.74,41.74
S$13973
  Bottom 0: 158.74,41.74 159.09,41.73
S$13974
  Bottom 0: 159.09,41.73 159.3,41.76
S$13975
  Bottom 0: 159.3,41.76 153.04,35.51
S$13976
  Bottom 0: 153.04,35.51 150.53,35.51
S$13977
  Bottom 0: 148.77,36.7 148.83,36.8
S$13978
  Bottom 0: 148.83,36.8 148.88,37.05
S$13979
  Bottom 0: 148.88,37.05 148.83,37.3
S$13980
  Bottom 0: 148.83,37.3 148.7,37.51
S$13981
  Bottom 0: 148.7,37.51 148.5,37.66
S$13982
  Bottom 0: 148.5,37.66 148.25,37.73
S$13983
  Bottom 0: 148.25,37.73 148,37.71
S$13984
  Bottom 0: 148,37.71 147.78,37.59
S$13985
  Bottom 0: 147.78,37.59 147.61,37.41
S$13986
  Bottom 0: 147.61,37.41 147.52,37.17
S$13987
  Bottom 0: 147.52,37.17 147.52,37
S$13988
  Bottom 0: 147.52,37 147.5,36.99
S$13989
  Bottom 0: 147.5,36.99 147.5,40.98
S$13990
  Bottom 0: 147.5,40.98 153.1,46.58
S$13991
  Bottom 0: 153.1,46.58 153.08,46.53
S$13992
  Bottom 0: 153.08,46.53 152.95,46.1
S$13993
  Bottom 0: 152.95,46.1 152.91,45.66
S$13994
  Bottom 0: 152.91,45.66 152.95,45.21
S$13995
  Bottom 0: 152.95,45.21 153.08,44.78
S$13996
  Bottom 0: 153.08,44.78 153.29,44.39
S$13997
  Bottom 0: 153.29,44.39 153.58,44.04
S$13998
  Bottom 0: 153.58,44.04 153.92,43.76
S$13999
  Bottom 0: 153.92,43.76 154.31,43.54
S$14000
  Bottom 0: 154.31,43.54 154.74,43.42
S$14001
  Bottom 0: 154.74,43.42 155.19,43.37
S$14002
  Bottom 0: 155.19,43.37 155.64,43.42
S$14003
  Bottom 0: 155.64,43.42 156.06,43.54
S$14004
  Bottom 0: 156.06,43.54 156.46,43.76
S$14005
  Bottom 0: 156.46,43.76 156.81,44.04
S$14006
  Bottom 0: 156.81,44.04 156.98,44.26
S$14007
  Bottom 0: 156.98,44.26 156.98,43.4
S$14008
  Bottom 0: 156.98,43.4 154.03,40.44
S$14009
  Bottom 0: 154.03,40.44 154.05,40.58
S$14010
  Bottom 0: 154.05,40.58 154,40.92
S$14011
  Bottom 0: 154,40.92 153.87,41.25
S$14012
  Bottom 0: 153.87,41.25 153.67,41.53
S$14013
  Bottom 0: 153.67,41.53 153.4,41.76
S$14014
  Bottom 0: 153.4,41.76 153.08,41.91
S$14015
  Bottom 0: 153.08,41.91 152.74,41.97
S$14016
  Bottom 0: 152.74,41.97 152.39,41.95
S$14017
  Bottom 0: 152.39,41.95 152.06,41.84
S$14018
  Bottom 0: 152.06,41.84 151.76,41.65
S$14019
  Bottom 0: 151.76,41.65 151.52,41.4
S$14020
  Bottom 0: 151.52,41.4 151.35,41.09
S$14021
  Bottom 0: 151.35,41.09 151.26,40.75
S$14022
  Bottom 0: 151.26,40.75 151.26,40.4
S$14023
  Bottom 0: 151.26,40.4 151.35,40.06
S$14024
  Bottom 0: 151.35,40.06 151.52,39.75
S$14025
  Bottom 0: 151.52,39.75 151.76,39.5
S$14026
  Bottom 0: 151.76,39.5 152.06,39.31
S$14027
  Bottom 0: 152.06,39.31 152.39,39.2
S$14028
  Bottom 0: 152.39,39.2 152.74,39.19
S$14029
  Bottom 0: 152.74,39.19 152.78,39.19
S$14030
  Bottom 0: 152.78,39.19 152.12,38.53
S$14031
  Bottom 0: 152.12,38.53 150.79,38.53
S$14032
  Bottom 0: 150.79,38.53 150.72,38.53
S$14033
  Bottom 0: 150.72,38.53 150.66,38.51
S$14034
  Bottom 0: 150.66,38.51 150.59,38.49
S$14035
  Bottom 0: 150.59,38.49 150.53,38.45
S$14036
  Bottom 0: 150.53,38.45 150.48,38.41
S$14037
  Bottom 0: 150.48,38.41 148.77,36.7
S$14038
  Bottom 0: 146.6,41.67 146.65,41.78
S$14039
  Bottom 0: 146.65,41.78 146.69,42.08
S$14040
  Bottom 0: 146.69,42.08 146.65,42.38
S$14041
  Bottom 0: 146.65,42.38 146.51,42.65
S$14042
  Bottom 0: 146.51,42.65 146.31,42.87
S$14043
  Bottom 0: 146.31,42.87 146.05,43.02
S$14044
  Bottom 0: 146.05,43.02 145.75,43.09
S$14045
  Bottom 0: 145.75,43.09 145.6,43.08
S$14046
  Bottom 0: 145.6,43.08 150.41,47.89
S$14047
  Bottom 0: 150.41,47.89 150.44,47.94
S$14048
  Bottom 0: 150.44,47.94 150.49,48
S$14049
  Bottom 0: 150.49,48 150.51,48.06
S$14050
  Bottom 0: 150.51,48.06 150.53,48.13
S$14051
  Bottom 0: 150.53,48.13 150.53,48.2
S$14052
  Bottom 0: 150.53,48.2 150.53,53.19
S$14053
  Bottom 0: 150.53,53.19 150.71,53.02
S$14054
  Bottom 0: 150.71,53.02 151,52.87
S$14055
  Bottom 0: 151,52.87 151.32,52.8
S$14056
  Bottom 0: 151.32,52.8 151.65,52.82
S$14057
  Bottom 0: 151.65,52.82 151.86,52.9
S$14058
  Bottom 0: 151.86,52.9 152.92,51.85
S$14059
  Bottom 0: 152.92,51.85 152.88,51.83
S$14060
  Bottom 0: 152.88,51.83 152.83,51.77
S$14061
  Bottom 0: 152.83,51.77 152.79,51.7
S$14062
  Bottom 0: 152.79,51.7 152.78,51.63
S$14063
  Bottom 0: 152.78,51.63 152.78,49.85
S$14064
  Bottom 0: 152.78,49.85 152.79,49.77
S$14065
  Bottom 0: 152.79,49.77 152.83,49.7
S$14066
  Bottom 0: 152.83,49.7 152.88,49.64
S$14067
  Bottom 0: 152.88,49.64 152.96,49.6
S$14068
  Bottom 0: 152.96,49.6 153.03,49.59
S$14069
  Bottom 0: 153.03,49.59 154.52,49.59
S$14070
  Bottom 0: 154.52,49.59 146.6,41.67
S$14071
  Bottom 0: 236.58,42.96 236.6,43.12
S$14072
  Bottom 0: 236.6,43.12 236.55,43.46
S$14073
  Bottom 0: 236.55,43.46 236.43,43.79
S$14074
  Bottom 0: 236.43,43.79 236.22,44.07
S$14075
  Bottom 0: 236.22,44.07 235.95,44.3
S$14076
  Bottom 0: 235.95,44.3 235.63,44.45
S$14077
  Bottom 0: 235.63,44.45 235.29,44.51
S$14078
  Bottom 0: 235.29,44.51 234.94,44.49
S$14079
  Bottom 0: 234.94,44.49 234.61,44.38
S$14080
  Bottom 0: 234.61,44.38 234.31,44.19
S$14081
  Bottom 0: 234.31,44.19 234.07,43.94
S$14082
  Bottom 0: 234.07,43.94 233.9,43.63
S$14083
  Bottom 0: 233.9,43.63 233.89,43.56
S$14084
  Bottom 0: 233.89,43.56 232.3,43.56
S$14085
  Bottom 0: 232.3,43.56 232.66,43.76
S$14086
  Bottom 0: 232.66,43.76 233,44.04
S$14087
  Bottom 0: 233,44.04 233.29,44.39
S$14088
  Bottom 0: 233.29,44.39 233.5,44.78
S$14089
  Bottom 0: 233.5,44.78 233.63,45.21
S$14090
  Bottom 0: 233.63,45.21 233.68,45.66
S$14091
  Bottom 0: 233.68,45.66 233.63,46.1
S$14092
  Bottom 0: 233.63,46.1 233.5,46.53
S$14093
  Bottom 0: 233.5,46.53 233.29,46.93
S$14094
  Bottom 0: 233.29,46.93 233,47.27
S$14095
  Bottom 0: 233,47.27 232.66,47.56
S$14096
  Bottom 0: 232.66,47.56 232.26,47.77
S$14097
  Bottom 0: 232.26,47.77 231.84,47.89
S$14098
  Bottom 0: 231.84,47.89 231.39,47.94
S$14099
  Bottom 0: 231.39,47.94 230.94,47.89
S$14100
  Bottom 0: 230.94,47.89 230.52,47.77
S$14101
  Bottom 0: 230.52,47.77 230.12,47.56
S$14102
  Bottom 0: 230.12,47.56 229.78,47.27
S$14103
  Bottom 0: 229.78,47.27 229.49,46.93
S$14104
  Bottom 0: 229.49,46.93 229.28,46.53
S$14105
  Bottom 0: 229.28,46.53 229.15,46.1
S$14106
  Bottom 0: 229.15,46.1 229.1,45.66
S$14107
  Bottom 0: 229.1,45.66 229.15,45.21
S$14108
  Bottom 0: 229.15,45.21 229.28,44.78
S$14109
  Bottom 0: 229.28,44.78 229.49,44.39
S$14110
  Bottom 0: 229.49,44.39 229.78,44.04
S$14111
  Bottom 0: 229.78,44.04 230.12,43.76
S$14112
  Bottom 0: 230.12,43.76 230.48,43.56
S$14113
  Bottom 0: 230.48,43.56 225.34,43.56
S$14114
  Bottom 0: 225.34,43.56 216.1,52.8
S$14115
  Bottom 0: 216.1,52.8 216.42,52.82
S$14116
  Bottom 0: 216.42,52.82 216.72,52.93
S$14117
  Bottom 0: 216.72,52.93 216.99,53.11
S$14118
  Bottom 0: 216.99,53.11 217.19,53.37
S$14119
  Bottom 0: 217.19,53.37 217.32,53.67
S$14120
  Bottom 0: 217.32,53.67 217.37,53.98
S$14121
  Bottom 0: 217.37,53.98 217.32,54.3
S$14122
  Bottom 0: 217.32,54.3 217.19,54.61
S$14123
  Bottom 0: 217.19,54.61 216.99,54.86
S$14124
  Bottom 0: 216.99,54.86 216.72,55.05
S$14125
  Bottom 0: 216.72,55.05 216.42,55.16
S$14126
  Bottom 0: 216.42,55.16 216.09,55.18
S$14127
  Bottom 0: 216.09,55.18 215.77,55.11
S$14128
  Bottom 0: 215.77,55.11 215.48,54.96
S$14129
  Bottom 0: 215.48,54.96 215.25,54.74
S$14130
  Bottom 0: 215.25,54.74 215.07,54.47
S$14131
  Bottom 0: 215.07,54.47 214.99,54.15
S$14132
  Bottom 0: 214.99,54.15 214.99,53.92
S$14133
  Bottom 0: 214.99,53.92 199.96,68.94
S$14134
  Bottom 0: 199.96,68.94 199.96,68.99
S$14135
  Bottom 0: 199.96,68.99 199.95,69.06
S$14136
  Bottom 0: 199.95,69.06 199.94,69.13
S$14137
  Bottom 0: 199.94,69.13 199.91,69.19
S$14138
  Bottom 0: 199.91,69.19 199.87,69.25
S$14139
  Bottom 0: 199.87,69.25 199.82,69.3
S$14140
  Bottom 0: 199.82,69.3 198.91,70.21
S$14141
  Bottom 0: 198.91,70.21 198.86,70.25
S$14142
  Bottom 0: 198.86,70.25 198.8,70.29
S$14143
  Bottom 0: 198.8,70.29 198.74,70.31
S$14144
  Bottom 0: 198.74,70.31 198.68,70.33
S$14145
  Bottom 0: 198.68,70.33 198.6,70.33
S$14146
  Bottom 0: 198.6,70.33 197.39,70.33
S$14147
  Bottom 0: 197.39,70.33 197.32,70.33
S$14148
  Bottom 0: 197.32,70.33 197.25,70.31
S$14149
  Bottom 0: 197.25,70.31 197.19,70.29
S$14150
  Bottom 0: 197.19,70.29 197.13,70.25
S$14151
  Bottom 0: 197.13,70.25 197.08,70.21
S$14152
  Bottom 0: 197.08,70.21 192.03,65.16
S$14153
  Bottom 0: 192.03,65.16 191.98,65.1
S$14154
  Bottom 0: 191.98,65.1 191.94,65.04
S$14155
  Bottom 0: 191.94,65.04 191.92,64.98
S$14156
  Bottom 0: 191.92,64.98 191.91,64.91
S$14157
  Bottom 0: 191.91,64.91 191.9,64.84
S$14158
  Bottom 0: 191.9,64.84 191.9,63.48
S$14159
  Bottom 0: 191.9,63.48 191.75,63.43
S$14160
  Bottom 0: 191.75,63.43 191.45,63.24
S$14161
  Bottom 0: 191.45,63.24 191.21,62.99
S$14162
  Bottom 0: 191.21,62.99 191.08,62.75
S$14163
  Bottom 0: 191.08,62.75 189.7,62.75
S$14164
  Bottom 0: 189.7,62.75 189.8,62.81
S$14165
  Bottom 0: 189.8,62.81 190.14,63.09
S$14166
  Bottom 0: 190.14,63.09 190.43,63.44
S$14167
  Bottom 0: 190.43,63.44 190.65,63.83
S$14168
  Bottom 0: 190.65,63.83 190.77,64.26
S$14169
  Bottom 0: 190.77,64.26 190.82,64.71
S$14170
  Bottom 0: 190.82,64.71 190.77,65.15
S$14171
  Bottom 0: 190.77,65.15 190.65,65.58
S$14172
  Bottom 0: 190.65,65.58 190.43,65.98
S$14173
  Bottom 0: 190.43,65.98 190.14,66.32
S$14174
  Bottom 0: 190.14,66.32 189.8,66.61
S$14175
  Bottom 0: 189.8,66.61 189.41,66.82
S$14176
  Bottom 0: 189.41,66.82 188.98,66.94
S$14177
  Bottom 0: 188.98,66.94 188.53,66.99
S$14178
  Bottom 0: 188.53,66.99 188.08,66.94
S$14179
  Bottom 0: 188.08,66.94 187.66,66.82
S$14180
  Bottom 0: 187.66,66.82 187.26,66.61
S$14181
  Bottom 0: 187.26,66.61 186.92,66.32
S$14182
  Bottom 0: 186.92,66.32 186.63,65.98
S$14183
  Bottom 0: 186.63,65.98 186.42,65.58
S$14184
  Bottom 0: 186.42,65.58 186.29,65.15
S$14185
  Bottom 0: 186.29,65.15 186.25,64.71
S$14186
  Bottom 0: 186.25,64.71 186.29,64.26
S$14187
  Bottom 0: 186.29,64.26 186.42,63.83
S$14188
  Bottom 0: 186.42,63.83 186.63,63.44
S$14189
  Bottom 0: 186.63,63.44 186.92,63.09
S$14190
  Bottom 0: 186.92,63.09 187.26,62.81
S$14191
  Bottom 0: 187.26,62.81 187.36,62.75
S$14192
  Bottom 0: 187.36,62.75 177.49,62.75
S$14193
  Bottom 0: 177.49,62.75 176.21,64.02
S$14194
  Bottom 0: 176.21,64.02 176.16,64.07
S$14195
  Bottom 0: 176.16,64.07 176.1,64.11
S$14196
  Bottom 0: 176.1,64.11 176.03,64.13
S$14197
  Bottom 0: 176.03,64.13 175.97,64.14
S$14198
  Bottom 0: 175.97,64.14 175.9,64.15
S$14199
  Bottom 0: 175.9,64.15 172.22,64.15
S$14200
  Bottom 0: 172.22,64.15 172.15,64.14
S$14201
  Bottom 0: 172.15,64.14 172.09,64.13
S$14202
  Bottom 0: 172.09,64.13 172.03,64.11
S$14203
  Bottom 0: 172.03,64.11 171.97,64.07
S$14204
  Bottom 0: 171.97,64.07 171.91,64.02
S$14205
  Bottom 0: 171.91,64.02 171.45,63.57
S$14206
  Bottom 0: 171.45,63.57 171.59,63.83
S$14207
  Bottom 0: 171.59,63.83 171.72,64.26
S$14208
  Bottom 0: 171.72,64.26 171.77,64.71
S$14209
  Bottom 0: 171.77,64.71 171.72,65.15
S$14210
  Bottom 0: 171.72,65.15 171.59,65.58
S$14211
  Bottom 0: 171.59,65.58 171.38,65.98
S$14212
  Bottom 0: 171.38,65.98 171.09,66.32
S$14213
  Bottom 0: 171.09,66.32 170.75,66.61
S$14214
  Bottom 0: 170.75,66.61 170.35,66.82
S$14215
  Bottom 0: 170.35,66.82 169.93,66.94
S$14216
  Bottom 0: 169.93,66.94 169.48,66.99
S$14217
  Bottom 0: 169.48,66.99 169.03,66.94
S$14218
  Bottom 0: 169.03,66.94 168.61,66.82
S$14219
  Bottom 0: 168.61,66.82 168.21,66.61
S$14220
  Bottom 0: 168.21,66.61 167.87,66.32
S$14221
  Bottom 0: 167.87,66.32 167.58,65.98
S$14222
  Bottom 0: 167.58,65.98 167.37,65.58
S$14223
  Bottom 0: 167.37,65.58 167.24,65.15
S$14224
  Bottom 0: 167.24,65.15 167.2,64.71
S$14225
  Bottom 0: 167.2,64.71 167.24,64.26
S$14226
  Bottom 0: 167.24,64.26 167.37,63.83
S$14227
  Bottom 0: 167.37,63.83 167.58,63.44
S$14228
  Bottom 0: 167.58,63.44 167.87,63.09
S$14229
  Bottom 0: 167.87,63.09 168.21,62.81
S$14230
  Bottom 0: 168.21,62.81 168.4,62.7
S$14231
  Bottom 0: 168.4,62.7 158.88,62.7
S$14232
  Bottom 0: 158.88,62.7 158.88,66.85
S$14233
  Bottom 0: 158.88,66.85 158.88,66.92
S$14234
  Bottom 0: 158.88,66.92 158.86,66.99
S$14235
  Bottom 0: 158.86,66.99 158.84,67.05
S$14236
  Bottom 0: 158.84,67.05 158.8,67.11
S$14237
  Bottom 0: 158.8,67.11 158.76,67.17
S$14238
  Bottom 0: 158.76,67.17 154.04,71.88
S$14239
  Bottom 0: 154.04,71.88 154.18,71.85
S$14240
  Bottom 0: 154.18,71.85 154.5,71.87
S$14241
  Bottom 0: 154.5,71.87 154.81,71.98
S$14242
  Bottom 0: 154.81,71.98 155.07,72.17
S$14243
  Bottom 0: 155.07,72.17 155.28,72.42
S$14244
  Bottom 0: 155.28,72.42 155.41,72.72
S$14245
  Bottom 0: 155.41,72.72 155.45,73.04
S$14246
  Bottom 0: 155.45,73.04 155.41,73.36
S$14247
  Bottom 0: 155.41,73.36 155.28,73.66
S$14248
  Bottom 0: 155.28,73.66 155.07,73.92
S$14249
  Bottom 0: 155.07,73.92 154.81,74.11
S$14250
  Bottom 0: 154.81,74.11 154.5,74.21
S$14251
  Bottom 0: 154.5,74.21 154.18,74.23
S$14252
  Bottom 0: 154.18,74.23 153.85,74.17
S$14253
  Bottom 0: 153.85,74.17 153.57,74.02
S$14254
  Bottom 0: 153.57,74.02 153.33,73.8
S$14255
  Bottom 0: 153.33,73.8 153.16,73.52
S$14256
  Bottom 0: 153.16,73.52 153.07,73.2
S$14257
  Bottom 0: 153.07,73.2 153.07,72.88
S$14258
  Bottom 0: 153.07,72.88 153.08,72.84
S$14259
  Bottom 0: 153.08,72.84 145.7,80.23
S$14260
  Bottom 0: 145.7,80.23 145.73,80.26
S$14261
  Bottom 0: 145.73,80.26 145.94,80.55
S$14262
  Bottom 0: 145.94,80.55 146.07,80.87
S$14263
  Bottom 0: 146.07,80.87 146.11,81.22
S$14264
  Bottom 0: 146.11,81.22 146.07,81.56
S$14265
  Bottom 0: 146.07,81.56 145.94,81.89
S$14266
  Bottom 0: 145.94,81.89 145.73,82.17
S$14267
  Bottom 0: 145.73,82.17 145.46,82.39
S$14268
  Bottom 0: 145.46,82.39 145.15,82.55
S$14269
  Bottom 0: 145.15,82.55 144.8,82.61
S$14270
  Bottom 0: 144.8,82.61 144.45,82.59
S$14271
  Bottom 0: 144.45,82.59 144.12,82.48
S$14272
  Bottom 0: 144.12,82.48 143.83,82.29
S$14273
  Bottom 0: 143.83,82.29 143.59,82.04
S$14274
  Bottom 0: 143.59,82.04 143.42,81.73
S$14275
  Bottom 0: 143.42,81.73 143.33,81.39
S$14276
  Bottom 0: 143.33,81.39 143.33,81.04
S$14277
  Bottom 0: 143.33,81.04 143.42,80.7
S$14278
  Bottom 0: 143.42,80.7 143.59,80.39
S$14279
  Bottom 0: 143.59,80.39 143.83,80.14
S$14280
  Bottom 0: 143.83,80.14 144.12,79.95
S$14281
  Bottom 0: 144.12,79.95 144.45,79.84
S$14282
  Bottom 0: 144.45,79.84 144.8,79.83
S$14283
  Bottom 0: 144.8,79.83 144.84,79.83
S$14284
  Bottom 0: 144.84,79.83 147.5,77.17
S$14285
  Bottom 0: 147.5,77.17 142.98,77.17
S$14286
  Bottom 0: 142.98,77.17 138.78,81.37
S$14287
  Bottom 0: 138.78,81.37 138.79,81.42
S$14288
  Bottom 0: 138.79,81.42 138.75,81.67
S$14289
  Bottom 0: 138.75,81.67 138.62,81.89
S$14290
  Bottom 0: 138.62,81.89 138.41,82.04
S$14291
  Bottom 0: 138.41,82.04 138.17,82.11
S$14292
  Bottom 0: 138.17,82.11 137.92,82.08
S$14293
  Bottom 0: 137.92,82.08 137.7,81.97
S$14294
  Bottom 0: 137.7,81.97 137.52,81.78
S$14295
  Bottom 0: 137.52,81.78 137.43,81.55
S$14296
  Bottom 0: 137.43,81.55 137.43,81.3
S$14297
  Bottom 0: 137.43,81.3 137.52,81.06
S$14298
  Bottom 0: 137.52,81.06 137.7,80.88
S$14299
  Bottom 0: 137.7,80.88 137.92,80.76
S$14300
  Bottom 0: 137.92,80.76 138.16,80.74
S$14301
  Bottom 0: 138.16,80.74 138.99,79.91
S$14302
  Bottom 0: 138.99,79.91 138.8,80.01
S$14303
  Bottom 0: 138.8,80.01 138.45,80.07
S$14304
  Bottom 0: 138.45,80.07 138.1,80.05
S$14305
  Bottom 0: 138.1,80.05 137.77,79.94
S$14306
  Bottom 0: 137.77,79.94 137.48,79.75
S$14307
  Bottom 0: 137.48,79.75 137.24,79.5
S$14308
  Bottom 0: 137.24,79.5 137.12,79.29
S$14309
  Bottom 0: 137.12,79.29 137.12,84.43
S$14310
  Bottom 0: 137.12,84.43 139.95,87.25
S$14311
  Bottom 0: 139.95,87.25 139.98,87.31
S$14312
  Bottom 0: 139.98,87.31 140.02,87.35
S$14313
  Bottom 0: 140.02,87.35 140.03,87.39
S$14314
  Bottom 0: 140.03,87.39 140.06,87.45
S$14315
  Bottom 0: 140.06,87.45 140.06,87.51
S$14316
  Bottom 0: 140.06,87.51 140.08,87.57
S$14317
  Bottom 0: 140.08,87.57 140.08,87.69
S$14318
  Bottom 0: 140.08,87.69 140.53,87.69
S$14319
  Bottom 0: 140.53,87.69 140.6,87.7
S$14320
  Bottom 0: 140.6,87.7 140.67,87.74
S$14321
  Bottom 0: 140.67,87.74 140.73,87.8
S$14322
  Bottom 0: 140.73,87.8 140.77,87.87
S$14323
  Bottom 0: 140.77,87.87 140.78,87.95
S$14324
  Bottom 0: 140.78,87.95 140.78,89.65
S$14325
  Bottom 0: 140.78,89.65 141.39,89.65
S$14326
  Bottom 0: 141.39,89.65 141.22,89.46
S$14327
  Bottom 0: 141.22,89.46 141.08,89.16
S$14328
  Bottom 0: 141.08,89.16 141.03,88.84
S$14329
  Bottom 0: 141.03,88.84 141.08,88.52
S$14330
  Bottom 0: 141.08,88.52 141.22,88.22
S$14331
  Bottom 0: 141.22,88.22 141.43,87.97
S$14332
  Bottom 0: 141.43,87.97 141.7,87.8
S$14333
  Bottom 0: 141.7,87.8 142.01,87.7
S$14334
  Bottom 0: 142.01,87.7 142.34,87.7
S$14335
  Bottom 0: 142.34,87.7 142.65,87.8
S$14336
  Bottom 0: 142.65,87.8 142.92,87.97
S$14337
  Bottom 0: 142.92,87.97 143.14,88.22
S$14338
  Bottom 0: 143.14,88.22 143.27,88.52
S$14339
  Bottom 0: 143.27,88.52 143.32,88.84
S$14340
  Bottom 0: 143.32,88.84 143.27,89.16
S$14341
  Bottom 0: 143.27,89.16 143.14,89.46
S$14342
  Bottom 0: 143.14,89.46 142.96,89.65
S$14343
  Bottom 0: 142.96,89.65 157.54,89.65
S$14344
  Bottom 0: 157.54,89.65 157.54,87.95
S$14345
  Bottom 0: 157.54,87.95 157.55,87.87
S$14346
  Bottom 0: 157.55,87.87 157.59,87.8
S$14347
  Bottom 0: 157.59,87.8 157.65,87.74
S$14348
  Bottom 0: 157.65,87.74 157.72,87.7
S$14349
  Bottom 0: 157.72,87.7 157.8,87.69
S$14350
  Bottom 0: 157.8,87.69 158.19,87.69
S$14351
  Bottom 0: 158.19,87.69 155.47,84.98
S$14352
  Bottom 0: 155.47,84.98 155.42,84.92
